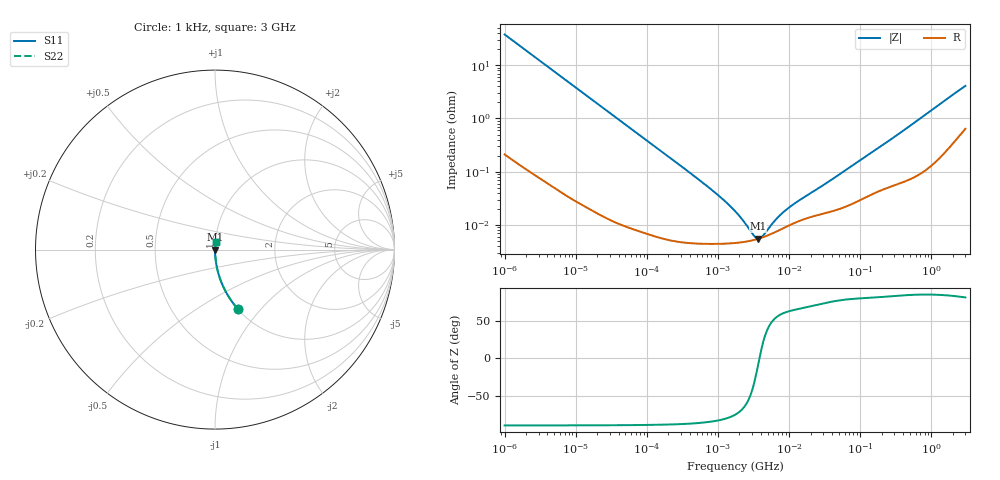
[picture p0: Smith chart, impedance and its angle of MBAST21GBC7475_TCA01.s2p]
! MBAST21GBC7475_TCA01  S-PARAMETER MODEL  ( Standard Model )
! Model Generated by TAIYO YUDEN Corporation (http://www.ty-top.com)
! Version 1.0
! TAIYO YUDEN Control No. 240819
! Copyright(c) 2024 TAIYO YUDEN CO.,LTD. All Rights Reserved.
! Product Description (link to TY-COMPAS)
! https://ds.yuden.co.jp/TYCOMPAS/or/detail?pn=MBAST21GBC7475KTCA01&u=M
! Products Name : Multilayer Ceramic Capacitors
! Characteristics :
!  Capacitance : 4.7 [uF] , Rated Voltage : 25 [V] , TCC : X7S
!  Case Size : 2.0 x 1.25 / 0.079 x 0.049 [mm/inch] , Thickness : 1.25 / 0.049 [mm/inch]
!  (Conditions: Temperature = 25 [degC] , DC Bias Voltage = 0 [V])
! External Node Assignments :
!  1  o---| |---o  2
! GND o---------o GND
! Frequency Range : 1kHz  -  3GHz  [ 401 STEP ]
# MHZ S RI R 50
! Freq[MHz].  S11 Real  S11 Imag  S21 Real  S21 Imag  S12 Real  S12 Imag  S22 Real  S22 Imag
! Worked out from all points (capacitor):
!   401 points, 1 kHz to 3 GHz, reference 50 ohm
!   read as one part in series: C = 4.19 uF near 1.077 kHz
!   lowest |Z| = 5.54 mohm at 3.651 MHz (marker M1)
!   series resonance near 3.823 MHz, so ESL is about 410 pH
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0.001  0.1272 -0.3304  0.8728 0.3304  0.8728 0.3304  0.1272 -0.3304
0.001685  0.0495 -0.2141  0.9505 0.2141  0.9505 0.2141  0.0495 -0.2141
0.00306  0.016 -0.1224  0.984 0.1224  0.984 0.1224  0.016 -0.1224
0.005768  0.00479 -0.0658  0.9952 0.0658  0.9952 0.0658  0.00479 -0.0658
0.01216  0.00123 -0.0314  0.9988 0.0314  0.9988 0.0314  0.00123 -0.0314
0.147855  6.46e-05 -0.00262  0.9999 0.00262  0.9999 0.00262  6.46e-05 -0.00262
0.791611  4.42e-05 -0.000469  1 0.000469  1 0.000469  4.42e-05 -0.000469
1.238299  4.45e-05 -0.00028  1 0.00028  1 0.00028  4.45e-05 -0.00028
1.732051  4.57e-05 -0.000177  1 0.000177  1 0.000177  4.57e-05 -0.000177
2.334012  4.79e-05 -0.000103  1 0.000103  1 0.000103  4.79e-05 -0.000103
2.514714  4.87e-05 -8.61e-05  1 8.61e-05  1 8.61e-05  4.87e-05 -8.61e-05
2.709407  4.96e-05 -6.99e-05  1 6.99e-05  1 6.99e-05  4.96e-05 -6.99e-05
3.651041  5.47e-05 -9e-06  0.9999 9e-06  0.9999 9e-06  5.47e-05 -9e-06
5.502215  6.7e-05 7.01e-05  0.9999 -7.01e-05  0.9999 -7.01e-05  6.7e-05 7.01e-05
5.928204  7e-05 8.45e-05  0.9999 -8.45e-05  0.9999 -8.45e-05  7e-05 8.45e-05
7.988506  8.48e-05 0.000143  0.9999 -0.000143  0.9999 -0.000143  8.48e-05 0.000143
9.991309  9.8e-05 0.000189  0.9999 -0.000189  0.9999 -0.000189  9.8e-05 0.000189
21.06097  0.000143 0.000387  0.9999 -0.000387  0.9999 -0.000387  0.000143 0.000387
41.2049  0.000183 0.000713  0.9998 -0.000713  0.9998 -0.000713  0.000183 0.000713
256.0921  0.000527 0.00384  0.9995 -0.00384  0.9995 -0.00384  0.000527 0.00384
1990.675  0.00411 0.0275  0.9959 -0.0275  0.9959 -0.0275  0.00411 0.0275
3000  0.00797 0.04  0.992 -0.04  0.992 -0.04  0.00797 0.04
